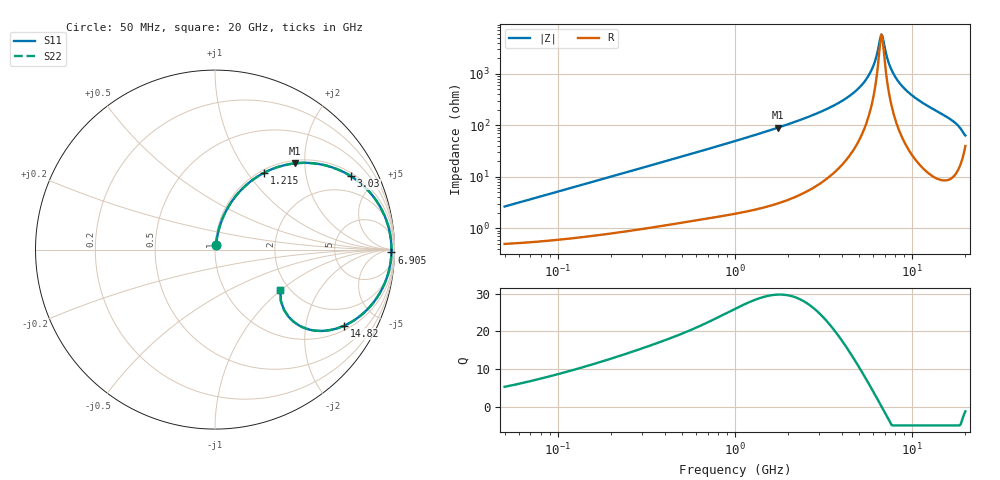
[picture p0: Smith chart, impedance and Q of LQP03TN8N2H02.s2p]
!Murata Part Number: LQP03TN8N2H02
!These Parameters are Measured in Series Mode Connection
!  o--[Z]--o
!Port1  Port2
!  o-------o
!Freq. Start=50[MHz] Stop=20[GHz], 401[Steps]
# Hz S RI R 50
!Freq.(Hz) S11(Real) S11(Imag) S21(Real) S21(Imag) S12(Real) S12(Imag) S22(Real) S22(Imag)
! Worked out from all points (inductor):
!   401 points, 50 MHz to 20 GHz, reference 50 ohm
!   read as one part in series: L = 8.21 nH near 51.52 MHz
!   highest Q = 29.7 at 1.741 GHz (marker M1), where L = 8.19 nH
!   self-resonance near 6.701 GHz
!   S11 on the Smith chart (normalised r, x): 50 MHz: 1.01, +0.05; 1.215 GHz: 1.04, +1.21; 3.03 GHz: 1.15, +3.63; 6.905 GHz: 62, -59; 14.82 GHz: 1.17, -3.27; 20 GHz: 1.79, -0.99
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5e7  0.00557 0.0256  0.9944 -0.0256  0.9944 -0.0256  0.00557 0.0256
1.364002e8  0.0113 0.0679  0.9887 -0.0679  0.9887 -0.0679  0.0113 0.0679
3.721004e8  0.0425 0.1745  0.9575 -0.1745  0.9575 -0.1745  0.0425 0.1745
1e9  0.2055 0.3853  0.7945 -0.3853  0.7945 -0.3853  0.2055 0.3853
1.214974e9  0.2755 0.4292  0.7245 -0.4292  0.7245 -0.4292  0.2755 0.4292
1.740566e9  0.4472 0.4807  0.5528 -0.4807  0.5528 -0.4807  0.4472 0.4807
2.728004e9  0.7026 0.4386  0.2974 -0.4386  0.2974 -0.4386  0.7026 0.4386
3.029571e9  0.7588 0.4079  0.2412 -0.4079  0.2412 -0.4079  0.7588 0.4079
4.087748e9  0.8916 0.2828  0.1084 -0.2828  0.1084 -0.2828  0.8916 0.2828
5.117541e9  0.9551 0.1623  0.0449 -0.1623  0.0449 -0.1623  0.9551 0.1623
5.944466e9  0.9775 0.0746  0.0225 -0.0746  0.0225 -0.0746  0.9775 0.0746
6.217679e9  0.9809 0.0476  0.0191 -0.0476  0.0191 -0.0476  0.9809 0.0476
6.601595e9  0.9832 0.0114  0.0168 -0.0114  0.0168 -0.0114  0.9832 0.0114
6.701223e9  0.9833 0.00226  0.0167 -0.00226  0.0167 -0.00226  0.9833 0.00226
6.905011e9  0.9831 -0.016  0.0169 0.016  0.0169 0.016  0.9831 -0.016
7.442007e9  0.9795 -0.0616  0.0205 0.0616  0.0205 0.0616  0.9795 -0.0616
8.141811e9  0.9693 -0.1161  0.0307 0.1161  0.0307 0.1161  0.9693 -0.1161
9.457416e9  0.9379 -0.2048  0.0621 0.2048  0.0621 0.2048  0.9379 -0.2048
1.149051e10  0.8683 -0.3121  0.1317 0.3121  0.1317 0.3121  0.8683 -0.3121
1.482269e10  0.718 -0.4246  0.282 0.4246  0.282 0.4246  0.718 -0.4246
1.800918e10  0.5105 -0.4412  0.4895 0.4412  0.4895 0.4412  0.5105 -0.4412
2e10  0.3634 -0.2263  0.6366 0.2263  0.6366 0.2263  0.3634 -0.2263
